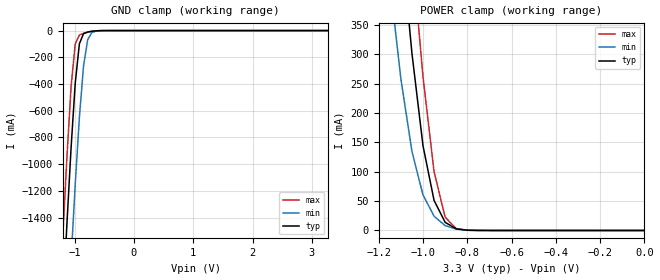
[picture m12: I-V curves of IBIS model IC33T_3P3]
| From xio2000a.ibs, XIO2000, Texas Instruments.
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|************************ IC33T @ 3.3V************************
[Model]   IC33T_3P3
Model_type   Input
Polarity   Non-Inverting
Vinh = 2.31V
Vinl = 0.99V
|   typ   min   max
C_comp   1.921pF   2.015pF   1.919pF
[Model Spec]
|   typ   min   max
Vinh   2.31V   2.10V   2.52V
Vinl   0.99V   0.90V   1.08V
[Temperature Range]   25   125   -40
[Voltage Range]   3.30V   3.00V   3.60V
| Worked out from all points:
|   GND clamp passes 1 mA (typ) near -0.59 V on its own axis
|   POWER clamp passes 1 mA (typ) near -0.81 V on its own axis
| (Vdd votage range)   1.50V   1.35V   1.65V
[GND_clamp]
| voltage   I(typ)   I(min)   I(max)
-3.3V     -22.44A    -23.22A    -22A
-1.2V     -2.054A    -2.928A    -1.544A
-1.13V    -1.446A    -2.31A     -946.6mA
-1.06V    -878mA     -1.714A    -422mA
-990mV    -393.9mA   -1.151A    -98.88mA
-920mV    -99.06mA   -650.3mA   -33.64mA
-850mV    -23.41mA   -265.9mA   -21.05mA
-780mV    -10.79mA   -67.97mA   -12.17mA
-710mV    -5.307mA   -14.65mA   -5.484mA
-640mV    -2.012mA   -4.071mA   -1.645mA
-430mV    -13.82uA   -80.66uA   -3.379uA
3.28V     115.7pA    2.974nA    91.57pA
[POWER_clamp]
| voltage   I(typ)   I(min)   I(max)
-3.3V     12.57A     11.67A     13.32A
-1.15V    728.1mA    424.8mA    974mA
-1.1V     502.9mA    258.7mA    718.5mA
-1.05V    302.1mA    134.9mA    477.1mA
-1V       144.4mA    60.62mA    262mA
-950mV    51.17mA    24.3mA     100.2mA
-900mV    13.92mA    8.343mA    22.77mA
-850mV    2.778mA    2.349mA    3.121mA
-800mV    440uA      584.7uA    298.1uA
-750mV    65.79uA    140uA      26.65uA
0V        117.5pA    2.521nA    104.5pA
